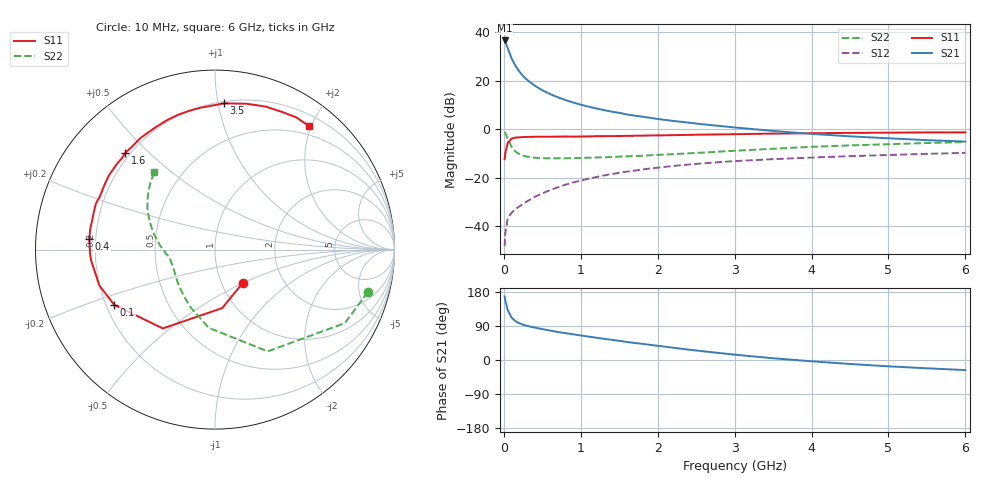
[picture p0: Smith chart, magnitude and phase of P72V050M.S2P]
! SIEMENS Small Signal Semiconductors
! BFP196
! Si NPN RF Bipolar Junction Transistor in SOT143
! VCE = 2 V  IC = 50 mA
! Common Emitter S-Parameters:  May  1996
# GHz  S  MA  R  50
!  f  S11  S21  S12  S22
! GHz  MAG  ANG  MAG  ANG  MAG  ANG  MAG  ANG
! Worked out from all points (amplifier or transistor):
!   36 points, 10 MHz to 6 GHz, reference 50 ohm
!   highest |S21| = 36.6 dB at 10 MHz (marker M1)
!   |S21| within 3 dB of that: start of sweep to 48.13 MHz
!   unconditionally stable (mu >= 1): 431.9 MHz to 4.395 GHz
!   at 250 MHz: K = 0.86, MSG = 26.3 dB, |S12| = -30.7 dB
!   at 1.4 GHz: K = 1.09, MAG = 11.0 dB, |S12| = -18.5 dB
!   at 6 GHz: K = 0.98, MSG = 2.3 dB, |S12| = -9.7 dB
!   S11 on the Smith chart (normalised r, x): 10 MHz: 1.25, -0.50; 100 MHz: 0.23, -0.24; 400 MHz: 0.17, +0.04; 1.6 GHz: 0.18, +0.43; 3.5 GHz: 0.21, +1.04; 6 GHz: 0.36, +1.96
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0.01  0.2417 -50.5  67.96 167.9  0.0039 79.9  0.8838 -15.5
0.02  0.3281 -82.9  63.21 155.8  0.0074 71.0  0.8315 -29.5
0.05  0.5268 -123.5  47.25 131.7  0.0145 54.9  0.6387 -62.6
0.1  0.6403 -151.3  29.21 112.1  0.019 48.5  0.4373 -94.5
0.15  0.6749 -162.8  20.49 102.8  0.0227 48.9  0.3504 -112.7
0.2  0.6819 -170.2  15.71 97.1  0.0256 52.3  0.3089 -124.8
0.25  0.6931 -175.1  12.57 93.1  0.0292 54.5  0.2859 -134.1
0.3  0.6966 -178.3  10.55 90.2  0.0326 56.9  0.2739 -140.1
0.4  0.7027 175.2  7.99 85.5  0.0404 60.2  0.2599 -149.1
0.5  0.7046 170.7  6.4 81.6  0.0477 62.0  0.2543 -155.1
0.6  0.7034 166.8  5.339 77.7  0.0558 62.6  0.2527 -159.1
0.7  0.7071 162.5  4.597 74.0  0.0638 63.1  0.2529 -162.1
0.9  0.7064 155.1  3.573 67.8  0.0803 61.8  0.2543 -166.7
1.1  0.7158 148.2  2.937 61.7  0.0959 60.4  0.26 -169.8
1.3  0.7227 141.6  2.494 55.9  0.112 57.8  0.2654 -172.8
1.6  0.7353 132.7  2.029 47.6  0.1343 53.7  0.2781 -176.5
2.2  0.7576 116.0  1.49 32.4  0.1757 45.1  0.3071 175.7
2.8  0.7864 100.6  1.176 18.5  0.2107 36.3  0.3474 166.5
3.5  0.8165 86.4  0.927 4.6  0.2428 26.3  0.398 156.3
4.5  0.8452 70.5  0.717 -10.5  0.2798 14.4  0.4663 143.8
5.5  0.8646 58.5  0.598 -21.9  0.3123 3.6  0.5217 133.3
6  0.8649 52.9  0.56 -26.6  0.327 -2.2  0.5476 128.1
